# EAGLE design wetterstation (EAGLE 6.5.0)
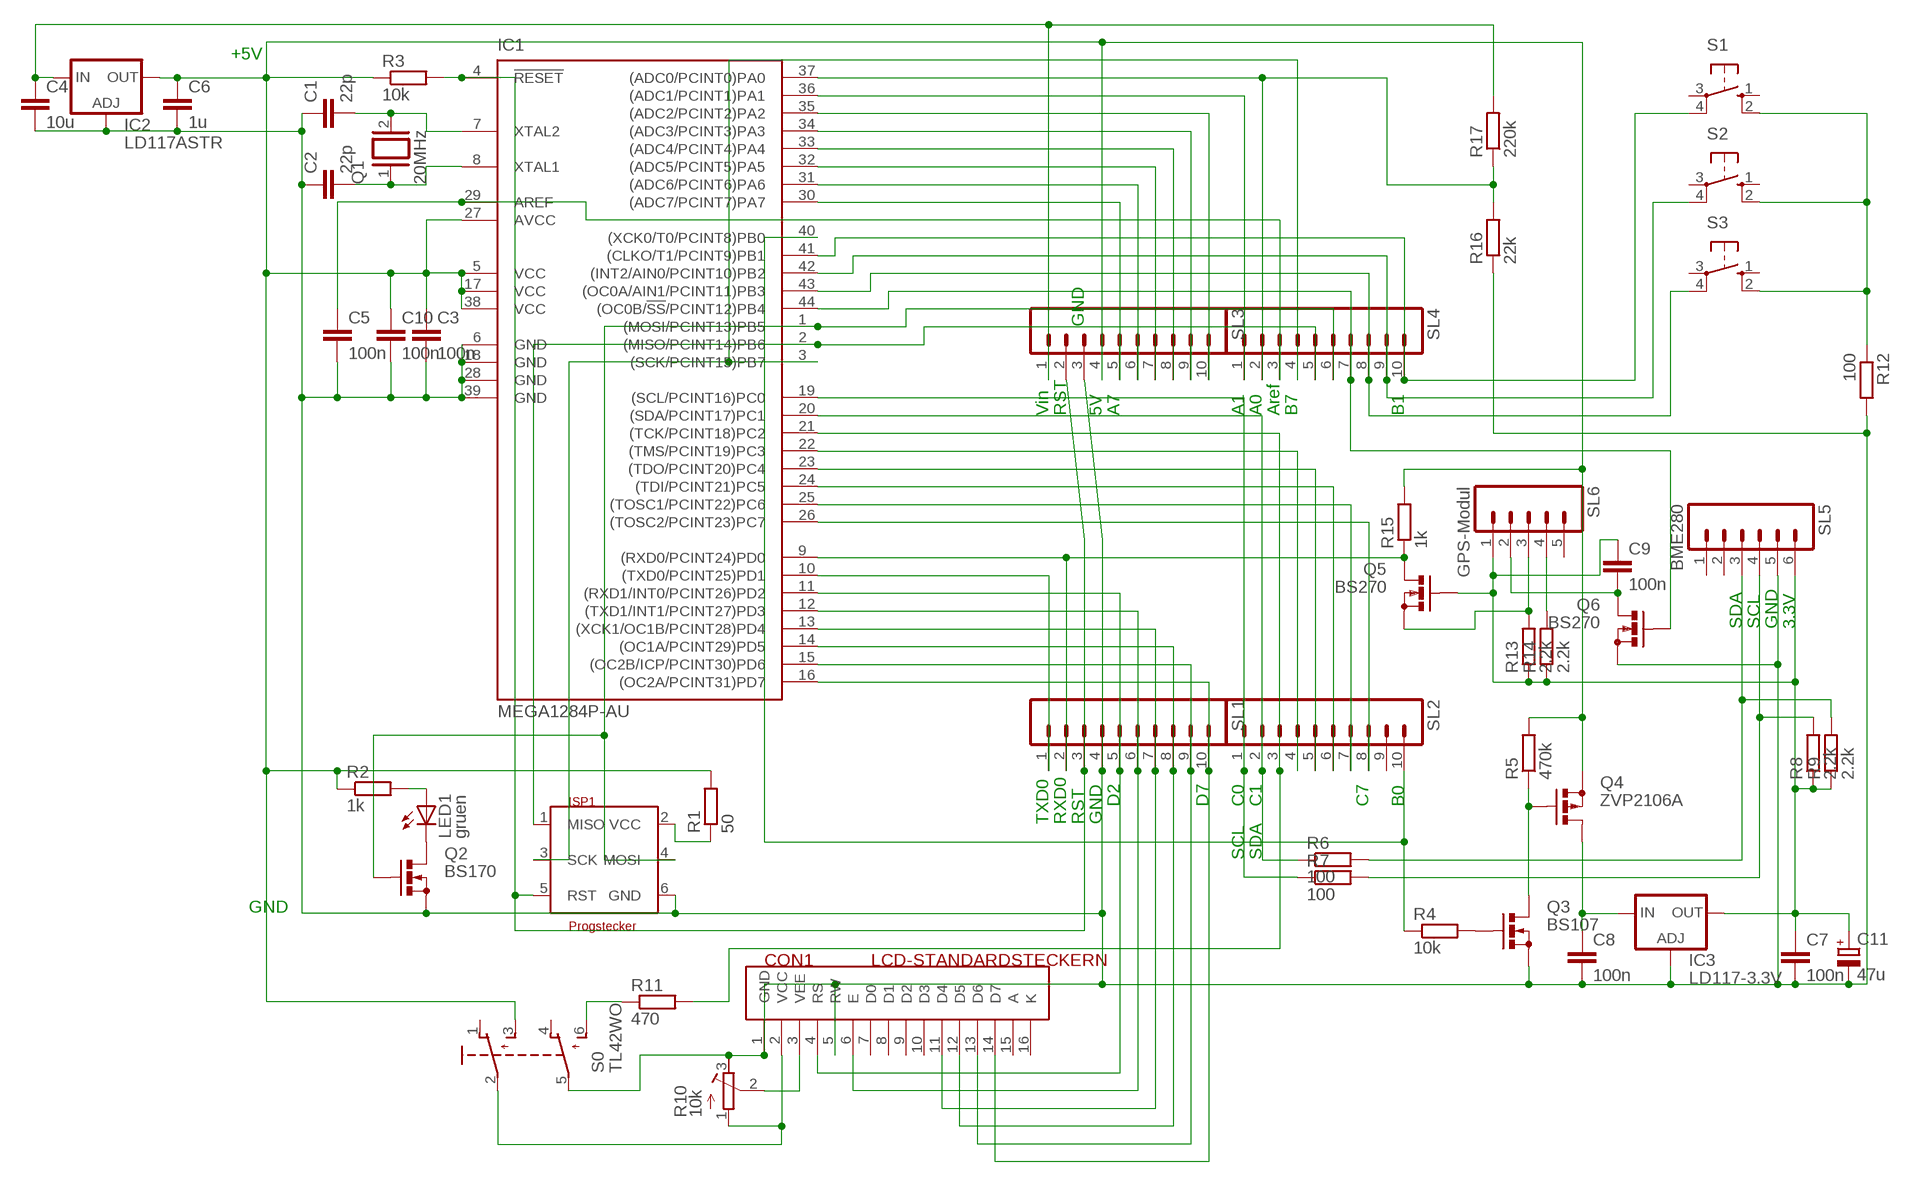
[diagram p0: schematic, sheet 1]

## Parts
C1  22p  C-EUC1206  [C1206]
C2  22p  C-EUC1206  [C1206]
C3  100n  C-EUC1206  [C1206]
C4  10u  C-EUC1206  [C1206]
C5  100n  C-EUC1206  [C1206]
C6  1u  C-EUC1206  [C1206]
C7  100n  C-EU025-025X050  [C025-025X050]
C8  100n  C-EU025-024X044  [C025-024X044]
C9  100n  C-EU025-024X044  [C025-024X044]
C10  100n  C-EUC1206  [C1206]
C11  47u  CPOL-EUE2-4  [E2-4]
CON1  LCD-STANDARDSTECKERN  [STECKER16]
IC1  MEGA1284P-AU  MEGA164P/324P/644P-AU  [TQFP44]
IC2  LD117ASTR  [SOT223]
IC3  LD117-3.3V  LD117ASTR  [SOT223]
ISP1  Progstecker  ISP6N  [ISP6]
LED1  gruen  LED3MM  [LED3MM]
Q1  20MHz  XTAL/S  [QS]
Q2  BS170  [SOT54E]
Q3  BS107  BS170  [SOT54E]
Q4  ZVP2106A  BS250  [SOT54E]
Q5  BS270  BS170  [SOT54E]
Q6  BS270  BS170  [SOT54E]
R1  50  R-EU_M1406  [M1406]
R2  1k  R-EU_M1406  [M1406]
R3  10k  R-EU_R3216  [R3216]
R4  10k  R-EU_0204/5  [0204/5]
R5  470k  R-EU_0204/5  [0204/5]
R6  100  R-EU_0204/5  [0204/5]
R7  100  R-EU_0204/5  [0204/5]
R8  2.2k  R-EU_0204/5  [0204/5]
R9  2.2k  R-EU_0204/5  [0204/5]
R10  10k  R-TRIMM64Z  [RTRIM64Z]
R11  470  R-EU_0204/5  [0204/5]
R12  100  R-EU_0204/5  [0204/5]
R13  2.2k  R-EU_0204/5  [0204/5]
R14  2.2k  R-EU_0204/5  [0204/5]
R15  1k  R-EU_0204/5  [0204/5]
R16  22k  R-EU_0204/5  [0204/5]
R17  220k  R-EU_0204/5  [0204/5]
S0  TL42WO  [TL4XWO]
S1  10-XX  [B3F-10XX]
S2  10-XX  [B3F-10XX]
S3  10-XX  [B3F-10XX]
SL1  M10  [10P]
SL2  M10  [10P]
SL3  M10  [10P]
SL4  M10  [10P]
SL5  BME280  M06  [06P]
SL6  GPS-Modul  M05  [05P]

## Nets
AREF: C5.1 IC1.29(AREF) SL4.3
GND [dick]: C1.1 C2.1 C3.2 C4.2 C5.2 C6.2 C7.2 C8.2 C10.2 C11.- CON1.1(GND) CON1.5(RW) IC1.6(GND) IC1.18(GND) IC1.28(GND) IC1.39(GND) IC2.1(ADJ) IC3.1(ADJ) ISP1.6(GND) Q2.S Q3.S Q6.S R10.3(E) R12.2 R16.1 S0.5(P1) SL1.4 SL3.3 SL5.5
N$1 [dick2]: C4.1 IC2.3(IN) R17.2 SL3.1
N$2: LED1.K(C) Q2.D
N$3: ISP1.2(VCC) R1.1
N$4: IC1.40((XCK0/T0/PCINT8)PB0) R4.1 SL2.10
N$5 [dick]: LED1.A R2.2
N$6: C2.2 IC1.8(XTAL1) Q1.1
N$7: IC1.3((SCK/PCINT15)PB7) ISP1.3(SCK) SL4.4
N$8: C1.2 IC1.7(XTAL2) Q1.2
N$9: IC1.10((TXD0/PCINT25)PD1) SL1.1
N$10: IC1.9((RXD0/PCINT24)PD0) Q5.D R15.1 SL1.2
N$11: IC1.2((MISO/PCINT14)PB6) ISP1.1(MISO) SL4.5
N$12: IC1.30((ADC7/PCINT7)PA7) SL3.5
N$13: IC1.31((ADC6/PCINT6)PA6) SL3.6
N$14: IC1.32((ADC5/PCINT5)PA5) SL3.7
N$15: IC1.33((ADC4/PCINT4)PA4) SL3.8
N$16: IC1.34((ADC3/PCINT3)PA3) SL3.9
N$17: IC1.35((ADC2/PCINT2)PA2) SL3.10
N$18: IC1.36((ADC1/PCINT1)PA1) SL4.1
N$19: IC1.37((ADC0/PCINT0)PA0) R16.2 R17.1 SL4.2
N$20: CON1.4(RS) IC1.11((RXD1/INT0/PCINT26)PD2) SL1.5
N$21: CON1.6(E) IC1.12((TXD1/INT1/PCINT27)PD3) SL1.6
N$22: CON1.11(D4) IC1.13((XCK1/OC1B/PCINT28)PD4) SL1.7
N$23: CON1.12(D5) IC1.14((OC1A/PCINT29)PD5) SL1.8
N$24: CON1.13(D6) IC1.15((OC2B/ICP/PCINT30)PD6) SL1.9
N$25: IC1.1((MOSI/PCINT13)PB5) ISP1.4(MOSI) Q2.G SL4.6
N$26: CON1.14(D7) IC1.16((OC2A/PCINT31)PD7) SL1.10
N$27: IC1.4(!RESET) ISP1.5(RST) R3.2 SL1.3 SL3.2
N$28: IC1.41((CLKO/T1/PCINT9)PB1) S1.4(P1) SL4.10
N$29: IC1.26((TOSC2/PCINT23)PC7) SL2.8
N$30: IC1.25((TOSC1/PCINT22)PC6) SL2.7
N$31: IC1.24((TDI/PCINT21)PC5) SL2.6
N$32: IC1.23((TDO/PCINT20)PC4) SL2.5
N$33: IC1.22((TMS/PCINT19)PC3) SL2.4
N$34: IC1.21((TCK/PCINT18)PC2) R11.2 SL2.3
N$35: IC1.20((SDA/PCINT17)PC1) R6.1 SL2.2
N$36: IC1.19((SCL/PCINT16)PC0) R7.1 SL2.1
N$37: IC1.42((INT2/AIN0/PCINT10)PB2) S2.4(P1) SL4.9
N$38: IC1.43((OC0A/AIN1/PCINT11)PB3) S3.4(P1) SL4.8
N$40: C7.1 C9.1 C11.+ IC3.4(OUT) Q5.G R8.1 R9.1 R13.1 R14.1 SL5.6 SL6.1
N$41: C8.1 IC3.3(IN) Q4.D
N$42: Q3.G R4.2
N$43: Q3.D Q4.G R5.1
N$44: R6.2 R9.2 SL5.3
N$45: R7.2 R8.2 SL5.4
N$46: CON1.3(VEE) R10.2(S)
N$47: CON1.2(VCC) R10.1(A) S0.2(P)
N$48: R11.1 S0.6(S1)
N$49 [dick]: C9.2 Q6.D SL6.2
N$50 [dick]: R12.1 S1.2(S1) S2.2(S1) S3.2(S1)
N$51: R14.2 SL6.4
N$52: Q5.S R13.2 SL6.3
N$53: IC1.44((OC0B/!SS!/PCINT12)PB4) Q6.G SL4.7
VCC [dick]: C3.1 C6.1 C10.1 IC1.5(VCC) IC1.17(VCC) IC1.27(AVCC) IC1.38(VCC) IC2.4(OUT) Q4.S R1.2 R2.1 R3.1 R5.2 R15.2 S0.3(S) SL3.4
Unconnected: CON1.7(D0) CON1.8(D1) CON1.9(D2) CON1.10(D3) CON1.15(A) CON1.16(K) S0.1(O) S0.4(O1) S1.1(S) S1.3(P) S2.1(S) S2.3(P) S3.1(S) S3.3(P) SL2.9 SL5.1 SL5.2 SL6.5

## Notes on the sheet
- +5V
- GND
- Vin | RST | 5V | A7 | A1 | A0 | Aref | B7 | B1
- SDA | SCL | GND | 3.3V
- D2 | D7 | C0 | C1 | C7 | B0
- TXD0 | RXD0 | RST | GND
- SCL | SDA
- GND

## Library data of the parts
C1-C10 = rcl:C-EU: CAPACITOR, European symbol
C11 = rcl:CPOL-EU: POLARIZED CAPACITOR, European symbol
CON1 = 6_stecker:LCD-STANDARDSTECKER: Standard-Stecker fuer die meisten LCD-Module
IC1 = avr-7:MEGA164P/324P/644P-AU
IC2 IC3 = v-reg:LD117A?*: Low drop fixed and adjustable positive voltage regulators 1 A Source: http://www.st.com/stonline/products/literature/ds/7194/ld1117axx.pdf
ISP1 = 6_stecker:ISP6: ISP-Stecker 6polig
LED1 = led:LED: LED
Q1 = special:XTAL/S: CRYSTAL
Q2 Q3 Q5 Q6 = transistor-small-signal:BS170: N-CHANNEL MOS FET
Q4 = transistor-small-signal:BS250: P-CHANNEL MOS FET
R1-R9 R11-R17 = rcl:R-EU_: RESISTOR, European symbol
R10 = rcl:R-TRIMM: Trimm resistor
S0 = switch:TL42WO: TINY SWITCH ON - MOM Source: http://www2.produktinfo.conrad.com/datenblaetter/700000-724999/705152-da-01-de-Subminiaturschalter_TL_36WO.pdf
S1-S3 = switch-omron:10-XX: OMRON SWITCH; MPN: B3F-1000; OC_FARNELL: 176432; OC_NEWARK: 36M3542
SL1-SL4 = con-amp-quick:M10: AMP QUICK CONNECTOR; OC_FARNELL: unknown; OC_NEWARK: unknown
SL5 = con-amp-quick:M06: AMP QUICK CONNECTOR; OC_FARNELL: unknown; OC_NEWARK: unknown
SL6 = con-amp-quick:M05: AMP QUICK CONNECTOR; OC_FARNELL: unknown; OC_NEWARK: unknown

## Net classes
1 dick: width 0.381 mm
2 dick2: width 0.762 mm

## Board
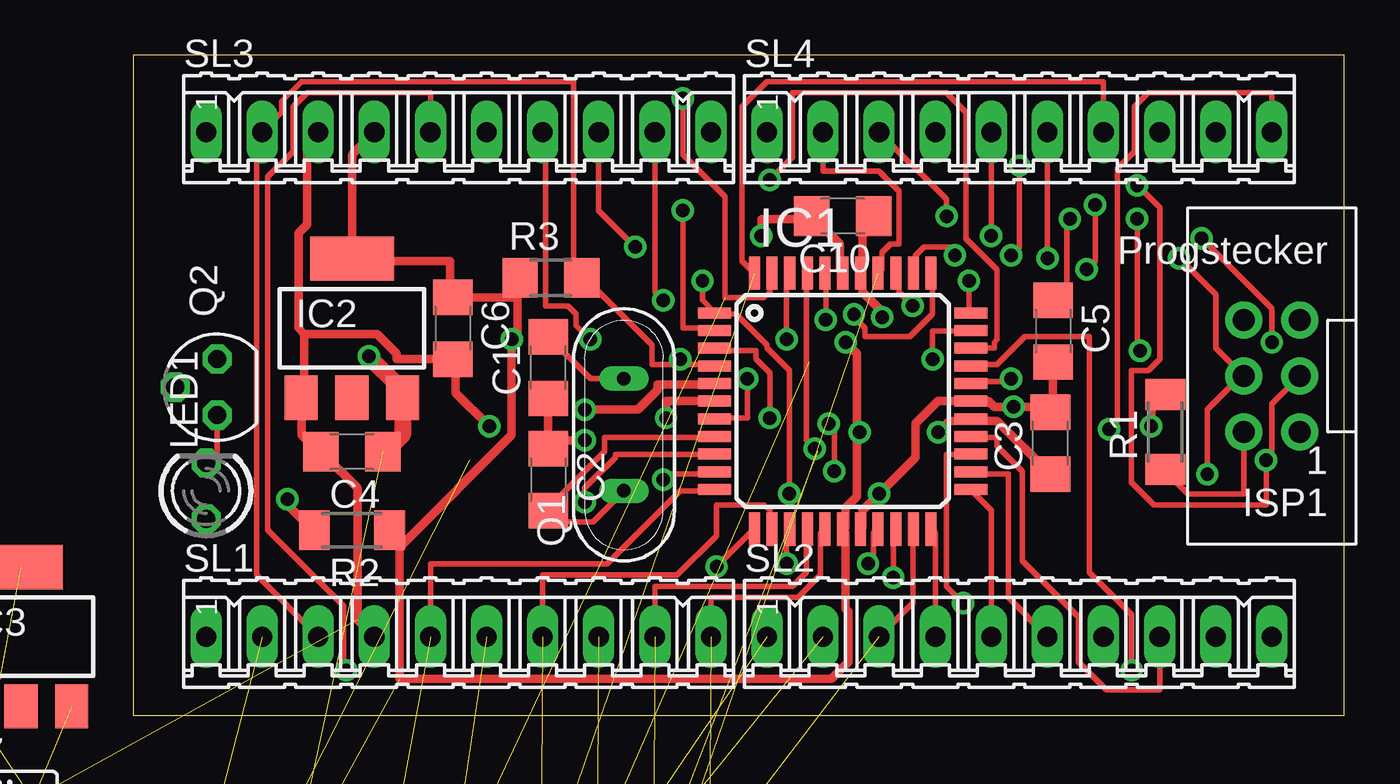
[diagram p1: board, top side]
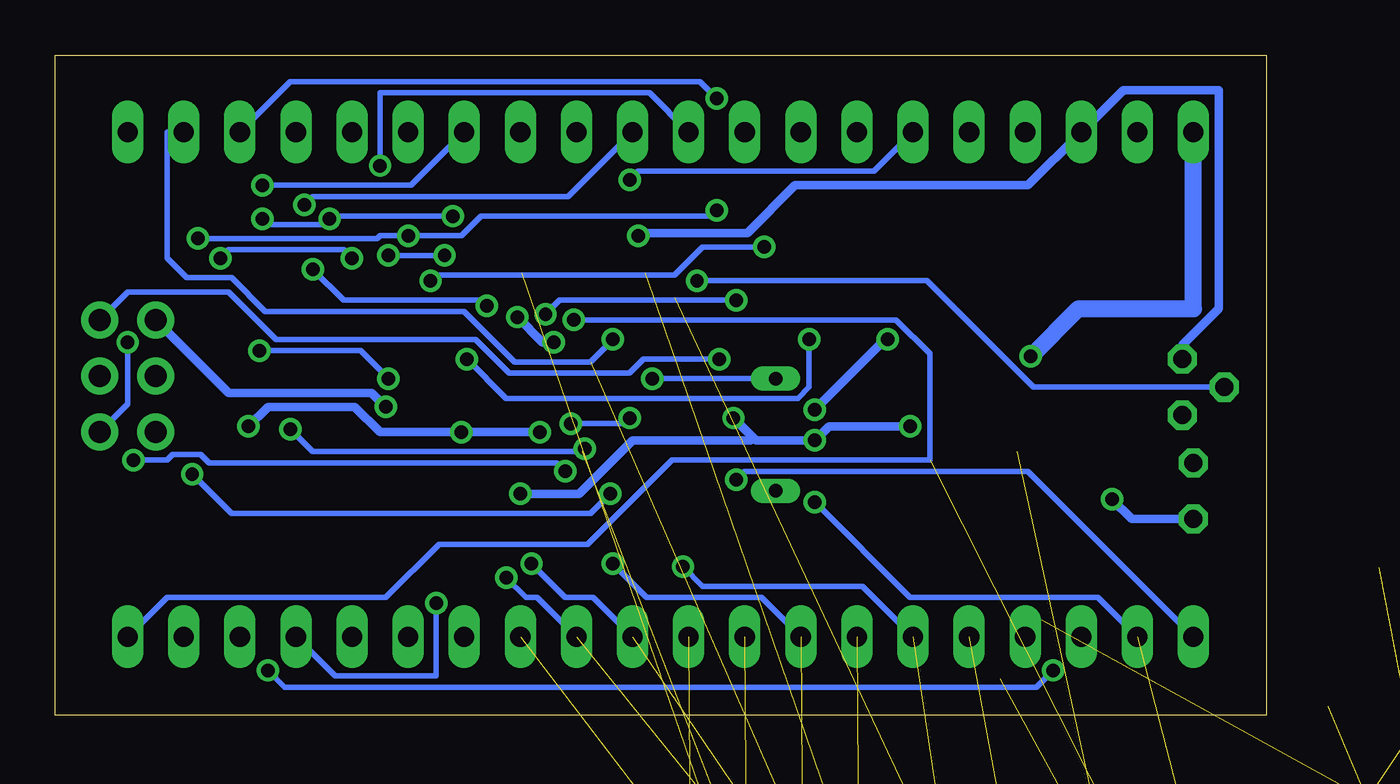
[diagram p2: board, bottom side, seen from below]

Size 54.84 x 29.9 mm. Coordinates in mm from the lower left corner, seen from the top.
Outline: 0,0 54.84,0 54.84,29.9 0,29.9 0,0
Copper layers (1*16): Top 0.035mm / dielectric 1.5mm / Bottom 0.035mm
Design rules "default": minimum track width 10mil, minimum drill 24mil, track to track 8mil, track to pad 8mil, pad to pad 8mil, via to via 8mil, smd to smd 8mil, copper to edge 40mil, drill to drill 8mil, minimum pad ring 10mil, minimum via ring 8mil, stop-mask expansion 4mil, vias tented up to drill 0mil, thermal gap 10mil

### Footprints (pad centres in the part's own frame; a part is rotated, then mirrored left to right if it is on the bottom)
C1206 = smd 1.6 x 1.8: 1 -1.4,0; 2 1.4,0
C025-025X050 = drill 0.813 octagon: 1 -1.27,0; 2 1.27,0
C025-024X044 = drill 0.813 octagon: 1 -1.27,0; 2 1.27,0
E2-4 = drill 0.813 pad 1.27: + -1.016,0 | drill 0.813 pad 1.27 octagon: - 1.016,0
STECKER16 = drill 1 long: 1 -17.78,0; 2 -15.24,0; 3 -12.7,0; 4 -10.16,0; 5 -7.62,0; 6 -5.08,0; 7 -2.54,0; 8 0,0; 9 2.54,0; 10 5.08,0; 11 7.62,0; 12 10.16,0; 13 12.7,0; 14 15.24,0; 15 17.78,0; 16 20.32,0
TQFP44 = smd 1.5 x 0.5: 1 -5.8,4; 2 -5.8,3.2; 3 -5.8,2.4; 4 -5.8,1.6; 5 -5.8,0.8; 6 -5.8,0; 7 -5.8,-0.8; 8 -5.8,-1.6; 9 -5.8,-2.4; 10 -5.8,-3.2; 11 -5.8,-4; 23 5.8,-4; 24 5.8,-3.2; 25 5.8,-2.4; 26 5.8,-1.6; 27 5.8,-0.8; 28 5.8,0; 29 5.8,0.8; 30 5.8,1.6; 31 5.8,2.4; 32 5.8,3.2; 33 5.8,4 | smd 0.5 x 1.5: 12 -4,-5.8; 13 -3.2,-5.8; 14 -2.4,-5.8; 15 -1.6,-5.8; 16 -0.8,-5.8; 17 0,-5.8; 18 0.8,-5.8; 19 1.6,-5.8; 20 2.4,-5.8; 21 3.2,-5.8; 22 4,-5.8; 34 4,5.8; 35 3.2,5.8; 36 2.4,5.8; 37 1.6,5.8; 38 0.8,5.8; 39 0,5.8; 40 -0.8,5.8; 41 -1.6,5.8; 42 -2.4,5.8; 43 -3.2,5.8; 44 -4,5.8
SOT223 = smd 1.5 x 2: 1 -2.3,-3.15; 2 0,-3.15; 3 2.3,-3.15 | smd 3.8 x 2: 4 0,3.15
ISP6 = drill 1 pad 1.676: 1 -1.27,2.54; 2 1.27,2.54; 3 -1.27,0; 4 1.27,0; 5 -1.27,-2.54; 6 1.27,-2.54
LED3MM = drill 0.813 octagon: A -1.27,0; K 1.27,0
QS = drill 0.61 long: 1 -2.54,0; 2 2.54,0
SOT54E = drill 0.813 octagon: D -1.27,0; G 0,1.905; S 1.27,0
M1406 = smd 1.4 x 1.8: 1 -1.7,0; 2 1.7,0
R3216 = smd 1.6 x 1.8: 1 -1.4,0; 2 1.4,0
0204/5 = drill 0.813 octagon: 1 -2.54,0; 2 2.54,0
RTRIM64Z = drill 0.61: 1 0,-2.54; 2 -2.54,0; 3 0,2.54
TL4XWO = drill 1.1 pad 1.422: 1 -2.54,-5.08; 2 0,-5.08; 3 2.54,-5.08; 4 -2.54,-6.985; 5 0,-6.985; 6 2.54,-6.985 | drill 1.1 pad 1.676: M1 -2.54,0; M2 2.54,0
B3F-10XX = drill 1.016 long: 1 -3.251,2.261; 2 3.251,2.261; 3 -3.251,-2.261; 4 3.251,-2.261
10P = drill 0.914 long: 1 -11.43,0; 2 -8.89,0; 3 -6.35,0; 4 -3.81,0; 5 -1.27,0; 6 1.27,0; 7 3.81,0; 8 6.35,0; 9 8.89,0; 10 11.43,0
06P = drill 0.914 long: 1 -6.35,0; 2 -3.81,0; 3 -1.27,0; 4 1.27,0; 5 3.81,0; 6 6.35,0
05P = drill 0.914 long: 1 -5.08,0; 2 -2.54,0; 3 0,0; 4 2.54,0; 5 5.08,0

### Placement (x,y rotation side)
C1  18.8,15.75 90 top
C2  18.8,10.67 270 top
C3  41.53,12.32 90 top
C4  9.91,11.94 180 top
C5  41.66,17.4 270 top
C6  14.48,17.53 270 top
C7  not placed on the board
C8  not placed on the board
C9  not placed on the board
C10  32.13,22.61 180 top
C11  not placed on the board
CON1  not placed on the board
IC1  32.13,14.22 0 top
IC2  9.91,17.53 0 top
IC3  -5.08,3.56 0 top
ISP1  51.56,15.37 180 top
LED1  3.3,10.16 90 top
Q1  22.23,12.7 90 top
Q2  3.81,14.86 90 top
Q3  not placed on the board
Q4  not placed on the board
Q5  not placed on the board
Q6  not placed on the board
R1  46.74,12.83 90 top
R2  9.91,8.38 180 top
R3  18.92,19.81 0 top
R4  not placed on the board
R5  not placed on the board
R6  not placed on the board
R7  not placed on the board
R8  not placed on the board
R9  not placed on the board
R10  not placed on the board
R11  not placed on the board
R12  not placed on the board
R13  not placed on the board
R14  not placed on the board
R15  not placed on the board
R16  not placed on the board
R17  not placed on the board
S0  not placed on the board
S1  not placed on the board
S2  not placed on the board
S3  not placed on the board
SL1  14.73,3.56 0 top
SL2  40.13,3.56 0 top
SL3  14.73,26.42 0 top
SL4  40.13,26.42 0 top
SL5  not placed on the board
SL6  not placed on the board

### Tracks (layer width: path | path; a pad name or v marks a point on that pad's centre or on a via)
AREF  (via drill 0.61)
  Top 0.254: v39.75,15.24 39.75,15.11 37.97,15.11 IC1.29 | v45.59,16.51 45.47,16.64 v45.47,22.48 | v42.42,22.48 42.29,22.35 42.29,19.56 41.66,18.92 C5.1 | SL4.3 36.83,23.37 v36.83,22.61
  Bottom 0.254: v39.75,15.24 41.02,16.51 v45.59,16.51 | v45.47,22.48 45.21,22.23 42.67,22.23 v42.42,22.48 42.29,22.61 v36.83,22.61
GND  (via drill 0.61)  (13 unrouted)
  Top 0.381: IC1.39 32.13,20.07 32,20.19 32,21.34 C10.2 30.61,22.48 28.45,22.48 v28.45,21.72 | C5.2 41.66,13.97 41.53,13.84 C3.2 41.4,13.97 v39.88,13.97 38.99,13.97 38.73,14.22 IC1.28 36.45,14.22 35.43,13.21 35.43,11.68 v33.78,10.03 33.02,9.27 33.02,8.51 IC1.18 | IC1.6 24.13,14.22 v24.13,13.46 | v20.45,12.45 18.8,12.45 C2.1 C1.1 | 7.75,17.27 11.05,17.27 11.94,16.38 11.94,16.13 C6.2 14.61,16 14.61,14.61 v16.13,13.08 | 7.75,17.27 7.75,14.48 IC2.1 7.62,14.35 7.62,12.7 8.38,11.94 C4.2 8.64,11.81 10.16,10.29 10.16,4.32 SL1.4 | SL3.3 7.87,25.91 7.87,22.23 7.49,21.84 7.49,17.53 7.75,17.27
  Bottom 0.381: Q2.S 3.81,16.76 2.16,18.41 2.16,28.32 6.48,28.32 SL3.3 10.79,24 21.34,24 23.5,21.84 28.32,21.84 v28.45,21.72 | ISP1.6 46.99,14.61 40.51,14.61 v39.88,13.97 | 23.24,12.57 23.11,12.45 v20.45,12.45 19.81,13.08 v16.13,13.08 | 23.24,12.57 v24.13,13.46 | v33.78,10.03 31.11,10.03 28.7,12.45 23.37,12.45 23.24,12.57
N$1  (via drill 0.61)  (1 unrouted)
  Top 0.762: C4.1 11.43,11.94 12.19,12.7 12.19,14.35 IC2.3 12.06,14.73 12.06,14.86 v10.67,16.26
  Bottom 0.762: SL3.1 3.3,18.41 8.51,18.41 v10.67,16.26
N$2
  Top 0.254: LED1.K 3.81,11.94 Q2.D
N$3
  Top 0.254: ISP1.2 50.29,10.03 47.75,10.03 46.74,11.05 R1.1
N$4  (via drill 0.61)  (1 unrouted)
  Top 0.254: v31.37,17.91 31.37,19.94 IC1.40
  Bottom 0.254: v31.37,17.91 16.76,17.91 15.24,16.38 15.24,11.56 26.92,11.56 30.73,7.75 37.47,7.75 39.88,5.33 49.78,5.33 SL2.10
N$5  (via drill 0.61)
  Top 0.381: v6.99,9.78 6.99,9.53 8.13,8.38 R2.2
  Bottom 0.381: v6.99,9.78 6.1,8.89 LED1.A
N$6
  Top 0.254: IC1.8 26.29,12.57 21.34,12.57 21.34,11.94 18.8,9.4 C2.2 18.8,8.76 20.83,8.76 Q1.1
N$7  (via drill 0.61)
  Top 0.254: v28.83,13.46 28.83,15.49 28.19,16.13 28.19,16.51 26.42,16.51 IC1.3 | v31.5,13.21 31.75,12.95 v31.75,11.05 | ISP1.3 51.56,14.1 51.56,11.81 v51.31,11.56 51.31,9.53 46.23,9.53 45.21,10.54 45.21,15.62 45.97,15.62 46.48,16.13 46.48,22.99 v45.47,24
  Bottom 0.254: v28.83,13.46 29.08,13.21 v31.5,13.21 | v31.75,11.05 32.13,11.43 47.88,11.43 48.26,11.81 49.53,11.81 49.78,11.56 v51.31,11.56 | SL4.4 38.73,24 v45.47,24
N$8  (via drill 0.61)
  Top 0.254: v27.81,15.24 27.81,13.46 26.42,13.46 IC1.7 | Q1.2 20.7,15.24 C1.2
  Bottom 0.254: Q1.2 v27.81,15.24
N$9  (via drill 0.61)
  Top 0.254: v24,10.67 24,10.92 26.29,10.92 IC1.10
  Bottom 0.254: v24,10.67 23.62,11.05 10.79,11.05 SL1.1
N$10  (via drill 0.61)  (2 unrouted)
  Top 0.254: v20.45,9.65 20.45,10.29 21.84,11.68 21.84,11.81 26.29,11.81 IC1.9
  Bottom 0.254: v20.45,9.65 16.13,5.33 7.62,5.33 SL1.2
N$11  (via drill 0.61)
  Top 0.254: v24.89,22.86 24.89,17.53 26.29,17.53 IC1.2 | SL4.5 v38.86,21.72 | v51.56,16.89 51.56,18.41 v48.39,21.59
  Bottom 0.254: v24.89,22.86 25.15,22.61 35.56,22.61 36.45,21.72 v38.86,21.72 40.13,21.72 40.26,21.59 v48.39,21.59 | ISP1.1 51.56,14.1 v51.56,16.89
N$12  (via drill 0.61)
  Top 0.254: v45.21,2.03 45.21,4.57 43.31,6.48 43.31,17.14 40.39,17.14 39.12,15.88 37.97,15.88 IC1.30 | v9.65,2.03 9.53,2.16 9.53,4.95 6.1,8.38 6.1,24.38 7.24,25.53 7.24,27.56 7.87,28.19 13.46,28.19 SL3.5
  Bottom 0.254: v45.21,2.03 44.45,1.27 10.41,1.27 v9.65,2.03
N$13  (via drill 0.61)
  Top 0.254: v28.83,24.26 29.84,25.27 29.84,28.19 36.83,28.19 37.72,27.3 37.72,21.59 39.12,20.19 39.12,17.02 38.99,16.89 38.99,16.64 37.97,16.64 IC1.31
  Bottom 0.254: v28.83,24.26 28.45,24.64 17.78,24.64 SL3.6
N$14  (via drill 0.61)
  Top 0.254: v36.2,16.13 36.2,17.4 37.85,17.4 IC1.32 | v20.7,17.02 20.07,17.65 20.07,18.16 19.68,18.54 18.67,18.54 18.67,26.29 SL3.7
  Bottom 0.254: v36.2,16.13 34.42,14.35 21.21,14.35 20.7,14.86 v20.7,17.02
N$15  (via drill 0.61)
  Top 0.254: v37.85,19.68 37.85,18.29 IC1.33 | v22.73,21.21 21.08,22.86 SL3.8
  Bottom 0.254: v37.85,19.68 37.59,19.94 26.8,19.94 25.53,21.21 v22.73,21.21
N$16  (via drill 0.61)
  Top 0.254: v32.64,18.16 32.64,18.03 33.15,17.53 33.15,17.14 35.18,17.14 36.2,18.16 36.2,19.94 IC1.34 | v24,18.8 23.62,19.18 SL3.9
  Bottom 0.254: v32.64,18.16 32,18.8 v24,18.8
N$17  (via drill 0.61)
  Top 0.254: v37.21,20.83 37.21,21.21 35.81,21.21 35.43,20.83 35.43,20.07 IC1.35 | v39.75,20.83 40.13,21.21 v40.13,24.89
  Bottom 0.254: v39.75,20.83 v37.21,20.83 | v40.13,24.89 40.13,28.19 27.94,28.19 SL3.10
N$18  (via drill 0.61)
  Top 0.254: v35.31,18.54 34.67,19.18 34.67,19.81 34.54,19.94 IC1.36 | v43.18,20.19 43.56,20.57 v43.56,23.11
  Bottom 0.254: v35.31,18.54 35.56,18.8 41.78,18.8 v43.18,20.19 | v43.56,23.11 43.18,23.5 31.62,23.5 SL4.1
N$19  (2 unrouted)
  Top 0.254: SL4.2 31.24,24.64 33.78,24.64 34.67,23.75 34.67,21.34 34.29,21.34 33.91,20.95 33.91,20.19 33.78,20.07 IC1.37
N$20  (1 unrouted)
  Top 0.254: SL1.5 13.46,6.86 21.46,6.86 24.77,10.16 26.29,10.16 IC1.11
N$21  (via drill 0.61)  (1 unrouted)
  Top 0.254: v26.42,6.73 28.07,8.38 IC1.12
  Bottom 0.254: v26.42,6.73 25.53,5.84 18.29,5.84 SL1.6
N$22  (1 unrouted)
  Top 0.254: SL1.7 18.54,6.35 24.64,6.35 26.42,8.13 26.42,9.53 28.57,9.53 28.83,9.27 28.83,8.51 IC1.13
N$23  (via drill 0.61)  (1 unrouted)
  Top 0.254: v29.59,6.86 29.59,8.26 29.72,8.38 IC1.14
  Bottom 0.254: v29.59,6.86 28.07,5.33 22.86,5.33 SL1.8
N$24  (1 unrouted)
  Top 0.254: SL1.9 23.62,5.84 29.84,5.84 30.48,6.48 30.48,8.38 IC1.15
N$25  (via drill 0.61)
  Top 0.254: v41.4,20.7 SL4.6 | v47.37,20.7 49.02,19.05 49.02,16.64 ISP1.4 50.16,15.37 48.64,13.84 v48.64,10.92 | v25.78,19.68 25.78,18.8 26.29,18.29 IC1.1 26.42,18.16 27.3,18.16 28.7,16.76 28.7,16.64 29.72,15.62 v29.72,10.03
  Bottom 0.254: v41.4,20.7 41.78,21.08 46.99,21.08 v47.37,20.7 | v25.78,19.68 15.37,19.68 10.54,14.86 Q2.G | v48.64,10.92 46.86,9.14 30.61,9.14 v29.72,10.03
N$26  (1 unrouted)
  Top 0.254: SL1.10 26.16,5.33 30.1,5.33 31.11,6.35 31.11,8.26 31.24,8.38 IC1.16
N$27  (via drill 0.61)
  Top 0.254: SL1.3 5.59,6.35 5.59,26.16 SL3.2 6.73,27.3 6.73,27.81 7.62,28.7 19.94,28.7 19.94,20.19 R3.2 20.45,19.81 23.5,16.76 23.5,15.88 24.77,15.88 | 24.77,15.88 26.29,15.88 IC1.4 | 24.77,15.88 v24.77,16.13
  Bottom 0.254: ISP1.5 51.56,19.18 46.99,19.18 44.83,17.02 35.81,17.02 34.29,15.49 28.83,15.49 28.19,16.13 v24.77,16.13
N$28  (via drill 0.61)  (1 unrouted)
  Top 0.254: v30.86,12.06 30.48,12.45 30.48,19.94 IC1.41 | v44.2,12.95 44.58,13.34 44.58,24.77 45.34,25.53 45.34,27.56 45.97,28.19 51.56,28.19 SL4.10
  Bottom 0.254: v30.86,12.06 30.99,11.94 43.18,11.94 v44.2,12.95
N$29
  Top 0.254: SL2.8 46.48,1.14 44.07,1.14 42.8,2.41 42.8,4.45 40.26,6.99 40.26,11.05 39.12,12.19 39.12,12.57 37.97,12.57 IC1.26
N$30  (via drill 0.61)
  Top 0.254: v37.59,5.08 36.83,5.84 36.83,11.81 37.85,11.81 IC1.25
  Bottom 0.254: v37.59,5.08 37.59,1.78 42.16,1.78 SL2.7
N$31
  Top 0.254: SL2.6 39.62,5.33 39.62,10.92 37.97,10.92 IC1.24
N$32
  Top 0.254: SL2.5 38.86,9.27 37.97,10.16 IC1.23
N$33
  Top 0.254: SL2.4 36.32,8.26 36.2,8.38 IC1.22
N$34  (1 unrouted)
  Top 0.254: SL2.3 35.31,5.08 35.31,8.38 IC1.21
N$35  (via drill 0.61)  (1 unrouted)
  Top 0.254: v34.42,6.22 34.42,8.38 IC1.20
  Bottom 0.254: v34.42,6.22 33.53,5.33 33.02,5.33 SL2.2
N$36  (via drill 0.61)  (1 unrouted)
  Top 0.254: v33.27,6.86 33.53,7.11 33.53,8.26 33.66,8.38 IC1.19
  Bottom 0.254: v33.27,6.86 31.75,5.33 30.48,5.33 SL2.1
N$37  (via drill 0.61)  (1 unrouted)
  Top 0.254: v29.59,17.02 29.59,19.81 29.72,19.94 IC1.42
  Bottom 0.254: v29.59,17.02 30.61,16 34.04,16 36.32,18.29 45.34,18.29 46.86,19.81 48.9,19.81 49.78,20.7 49.78,26.42 SL4.9
N$38  (via drill 0.61)  (1 unrouted)
  Top 0.254: v24.89,27.94 24.89,25.4 26.8,23.5 26.8,18.92 28.57,18.92 28.83,19.18 28.83,19.94 IC1.43
  Bottom 0.254: v24.89,27.94 25.65,28.7 44.2,28.7 SL4.8
N$40  (10 unrouted)
N$41  (2 unrouted)
N$42  (1 unrouted)
N$43  (2 unrouted)
N$44  (2 unrouted)
N$45  (2 unrouted)
N$46  (1 unrouted)
N$47  (2 unrouted)
N$48  (1 unrouted)
N$49  (2 unrouted)
N$50  (3 unrouted)
N$51  (1 unrouted)
N$52  (2 unrouted)
N$53  (1 unrouted)
  Top 0.254: SL4.7 43.94,28.7 28.7,28.7 27.56,27.56 27.56,20.57 28.07,20.07 IC1.44
VCC  (via drill 0.61)  (4 unrouted)
  Top 0.381: SL3.4 9.91,25.4 IC2.4 10.03,20.57 14.35,20.57 14.35,19.05 C6.1 17.27,18.92 R3.1 17.4,19.81 17.4,17.27 v17.14,17.02 17.14,12.7 12.19,7.75 R2.1 11.68,8.38 12.06,8 12.06,1.65 31.62,1.65 32.38,2.41 32.38,4.7 32.26,4.83 32.26,8.26 32.13,8.38 IC1.17 32.26,8.51 32.26,9.4 32.77,9.91 32.77,12.83 | v20.45,13.84 22.86,13.84 23.75,14.73 23.75,14.99 26.29,14.99 IC1.5 | C3.1 39.12,13.34 37.97,13.34 IC1.27 37.85,13.34 36.96,13.34 v36.45,12.83 | v46.1,13.08 46.1,13.84 46.74,14.48 R1.2 | C10.1 33.02,22.1 33.02,20.07 IC1.38 33.02,19.94 33.02,19.18 33.91,18.29 v33.91,18.03 | v32.26,16.89 32.77,16.38 32.77,12.83 | v32.89,12.83 32.77,12.83
  Bottom 0.381: v20.45,13.84 17.27,17.02 v17.14,17.02 | v46.1,13.08 45.21,13.97 41.27,13.97 40.13,12.83 v36.45,12.83 v32.89,12.83 | v33.91,18.03 32.77,16.89 v32.26,16.89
